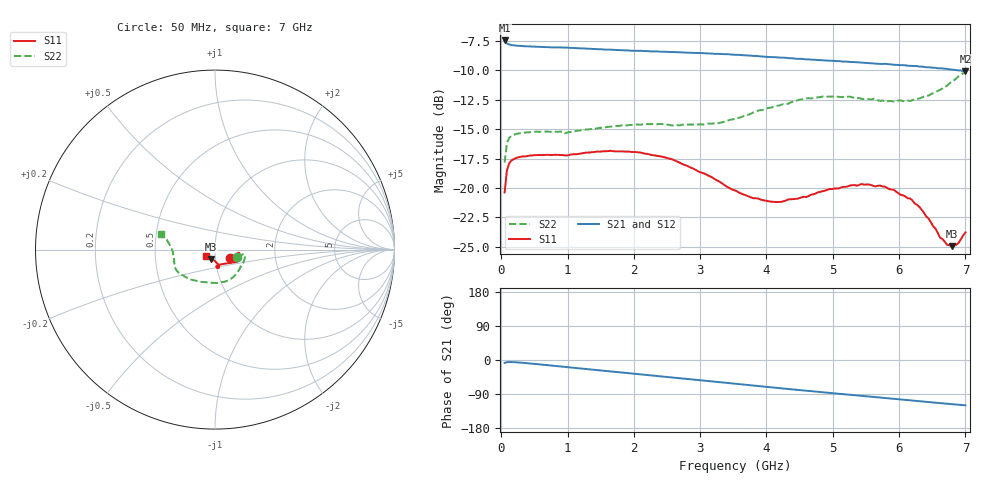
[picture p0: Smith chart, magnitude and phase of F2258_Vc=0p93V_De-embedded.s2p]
! Integrated Device Technology
! Corporate Headquarters
! 6024 Silver Creek Valley Road
! San Jose, CA 95138  USA
! Phone:  1-408-284-8200
! Toll Free:  1-800-223-1366
! Webpage:  http://www.idt.com/
! Timing and RF Division
! 515 Groton Road, Suite 102
! Westford, MA 01886-6024
! Device:  F2258
! Description: Voltage Variable RF Attenuator
! Frequency:  50.0 -  6000.00 MHz
! Package:  3x3 mm Thin QFN Plastic Package: 16 pin
! Ports:  2 RF, 2 DC
!  Pin  1  = NC
!  Pin  2  = NC
!  Pin  3  = RF2  = Port 2
!  Pin  4  = GND
!  Pin  5  = Vdd
!  Pin  6  = NC
!  Pin  7  = VCTRL
!  Pin  8  = NC
!  Pin  9  = GND
!  Pin 10  = RF1  = Port 1
!  Pin 11  = NC
!  Pin 12  = NC
!  Pin 13  = NC
!  Pin 14  = NC
!  Pin 15  = NC
!  Pin 16  = NC
! Vcntrl:  0.930 Volts
! Vdd:  +3.300 Volts
! Current:  1.152 mA
! Data:  The device was measured on a the F2258 evaluation board which has
!  individual transmission lines to the RF pins.  Data was collected
!  using a calibrated network analyzer.  The evaluation board was
!  de-embedded using a TRL calibration technique.
!  The reference plane is the edge of the package pin.
! Misc:  SN 10
!  Action Tracker AT0285
! Date Measured:  2014-12-10
! Date:  2016-01-13  MJV
! Note:
!  Integrated Device Technology supplies this data as a sample of measured
!  data at the package pin for this product.  Your particular data for this
!  product may vary.
!  Data was taken at 25 degrees C.
!  Integrated Device Technology reserves the right to change this data at anytime.
!Freq_(GHz)  S11M_(dB)  S11P_(deg)  S21M_(dB)  S21P_(deg)  S12M_(dB)  S12P_(deg)  S22M_(dB)  S22P_(deg)
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# GHz S dB R 50
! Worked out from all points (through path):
!   201 points, 50 MHz to 7 GHz, reference 50 ohm
!   highest |S21| = -7.48 dB at 50 MHz (marker M1); lowest = -10.1 dB at 7 GHz (marker M2)
!   group delay of S21, straight-line fit = 47 ps
!   lowest |S11| = -24.9 dB at 6.792 GHz (marker M3), VSWR 1.12, Z = 47.5 - j4.91 ohm
!   |S11| at or under -10 dB: start of sweep to end of sweep
!   |S22| runs from -17.8 to -10.1 dB; largest |S21 - S12| = 0.0027
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0.05  -20.38 -28.1  -7.48 -7.7  -7.49 -7.7  -17.84 -17.9
0.08475  -18.51 -13.5  -7.74 -5.8  -7.75 -5.8  -16.19 -10.1
0.1195  -17.90 -9.4  -7.82 -5.3  -7.83 -5.4  -15.74 -8.9
0.189  -17.55 -7.5  -7.90 -5.7  -7.92 -5.7  -15.48 -9.4
0.43225  -17.24 -9.0  -7.98 -9.1  -8.02 -9.2  -15.25 -15.8
0.9535  -17.23 -18.1  -8.08 -18.1  -8.11 -18.1  -15.36 -33.1
1.2315  -17.04 -21.1  -8.14 -22.9  -8.19 -22.9  -15.07 -41.7
1.6485  -16.84 -25.0  -8.26 -30.1  -8.29 -30.1  -14.80 -53.4
2.37825  -17.30 -30.1  -8.42 -42.5  -8.45 -42.5  -14.58 -73.3
3.0385  -18.72 -39.2  -8.55 -54.0  -8.57 -54.0  -14.61 -95.6
3.525  -20.21 -52.4  -8.69 -62.6  -8.70 -62.6  -14.13 -115.1
3.803  -20.88 -63.4  -8.79 -67.5  -8.78 -67.5  -13.58 -125.6
4.1505  -21.19 -74.7  -8.91 -73.5  -8.90 -73.5  -13.02 -136.1
4.7065  -20.53 -84.7  -9.11 -82.8  -9.10 -82.8  -12.37 -148.8
5.43625  -19.65 -81.2  -9.36 -94.6  -9.36 -94.6  -12.43 -160.6
5.85325  -20.10 -76.9  -9.49 -101.4  -9.51 -101.4  -12.62 -169.1
6.20075  -21.06 -77.2  -9.64 -107.1  -9.65 -107.0  -12.55 -177.6
6.444  -22.58 -82.6  -9.75 -110.9  -9.76 -110.9  -12.16 176.3
6.61775  -24.22 -92.9  -9.84 -113.7  -9.85 -113.7  -11.67 171.6
6.7915  -24.94 -114.4  -9.95 -116.5  -9.96 -116.5  -10.97 167.6
6.89575  -24.67 -129.4  -10.02 -118.1  -10.02 -118.1  -10.53 165.6
7  -23.77 -144.0  -10.08 -119.7  -10.07 -119.8  -10.06 163.6
